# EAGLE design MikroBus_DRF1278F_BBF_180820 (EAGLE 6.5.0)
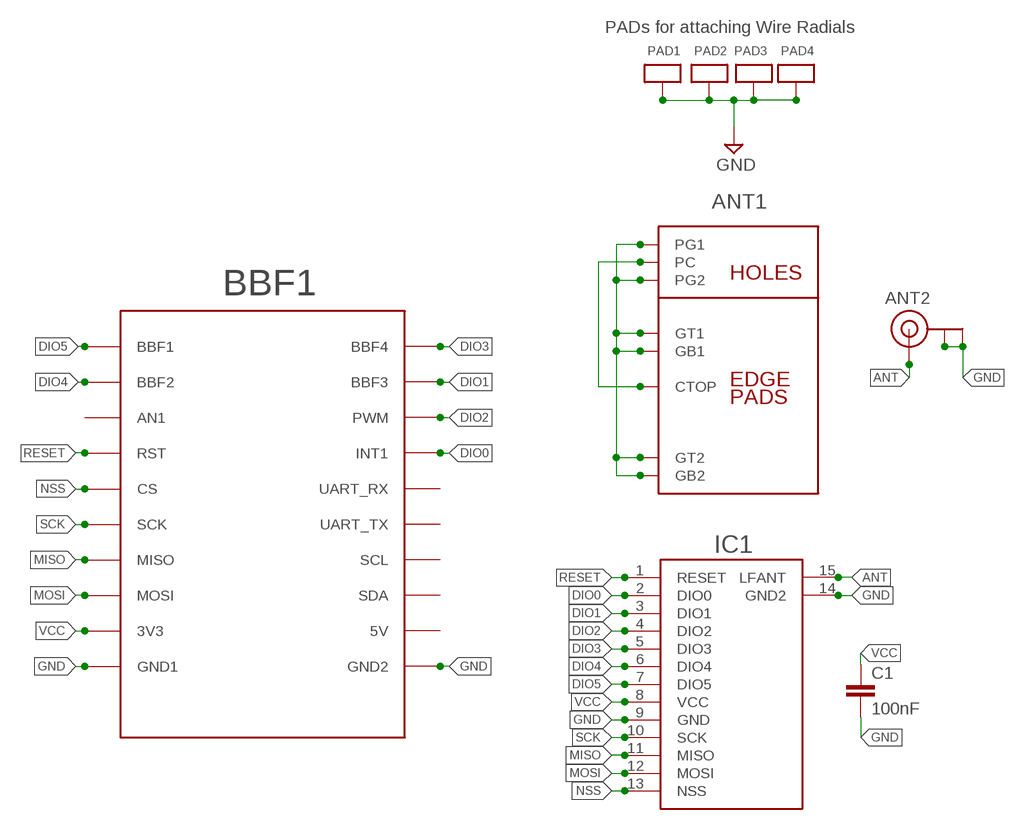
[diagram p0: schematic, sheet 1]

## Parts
ANT1  CUSTOMSMA  [CUSTOMSMA]
ANT2  ANTENNA_U.FL  [U.FL]
BBF1  BBFRIENDY2  [PCB_SOCKET_BBFRIENDLY2]
C1  100nF  C-EUC1206  [C1206]
IC1  DRF1278F  [DRF1278F]
PAD1  ANTPAD2  [ANTPAD2]
PAD2  ANTPAD2  [ANTPAD2]
PAD3  ANTPAD2  [ANTPAD2]
PAD4  ANTPAD2  [ANTPAD2]

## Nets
ANT: ANT1.CTOP ANT1.PC ANT2.3(SIGNAL) IC1.15(LFANT)
DIO0: BBF1.INT(INT1) IC1.2(DIO0)
DIO1: BBF1.BBF3 IC1.3(DIO1)
DIO2: BBF1.PWM IC1.4(DIO2)
DIO3: BBF1.BBF4 IC1.5(DIO3)
DIO4: BBF1.BBF2 IC1.6(DIO4)
DIO5: BBF1.BBF1 IC1.7(DIO5)
GND [VDD]: ANT1.G1 ANT1.G2 ANT1.GB1 ANT1.GB2 ANT1.GT1 ANT1.GT2 ANT2.1(GND) ANT2.2(GND) BBF1.GND1(GND2) BBF1.GND2(GND1) C1.2 IC1.9(GND) IC1.14(GND2) PAD1.P$1 PAD2.P$1 PAD3.P$1 PAD4.P$1
MISO: BBF1.MISO IC1.11(MISO)
MOSI: BBF1.MOSI IC1.12(MOSI)
NSS: BBF1.CS IC1.13(NSS)
RESET: BBF1.RST IC1.1(RESET)
SCK: BBF1.SCK IC1.10(SCK)
VCC [VDD]: BBF1.3V3 C1.1 IC1.8(VCC)
Unconnected: BBF1.5V BBF1.AN1 BBF1.RX(UART_RX) BBF1.SCL BBF1.SDA BBF1.TX(UART_TX)

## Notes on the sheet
- PADs for attaching Wire Radials
- BBF1

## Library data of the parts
ANT1 = con-coax:CUSTOMSMA
ANT2 = adafruit:ANTENNA_U.FL: U.FL Antenna Connector
BBF1 = My_Mikrobus:BBFRIENDY2
C1 = resistor:C-EU: CAPACITOR, European symbol
IC1 = LMA2:DRF1278F
PAD1-PAD4 = LMA2:ANTPAD2

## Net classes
0 default: width 0.152 mm
1 POWER: width 0.635 mm
2 VDD: width 0.635 mm

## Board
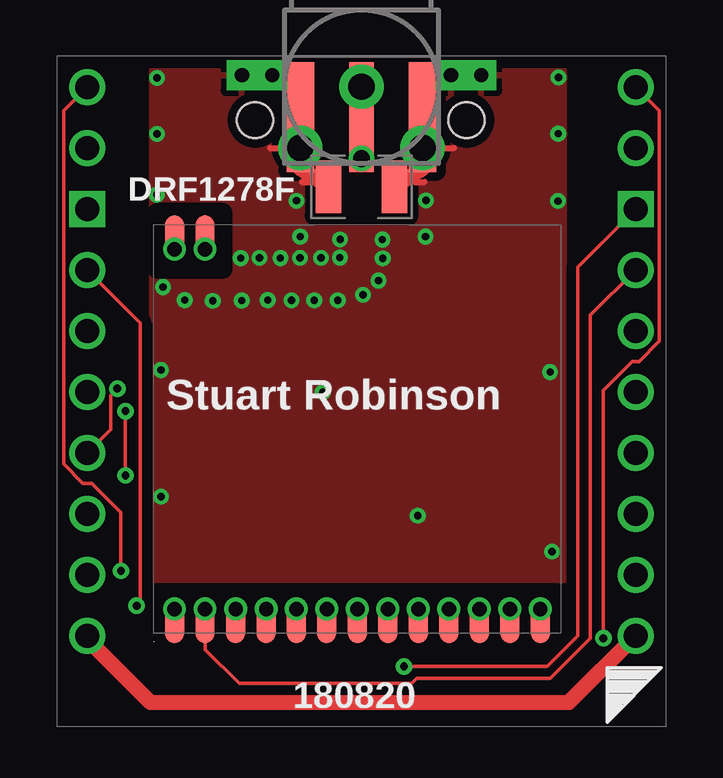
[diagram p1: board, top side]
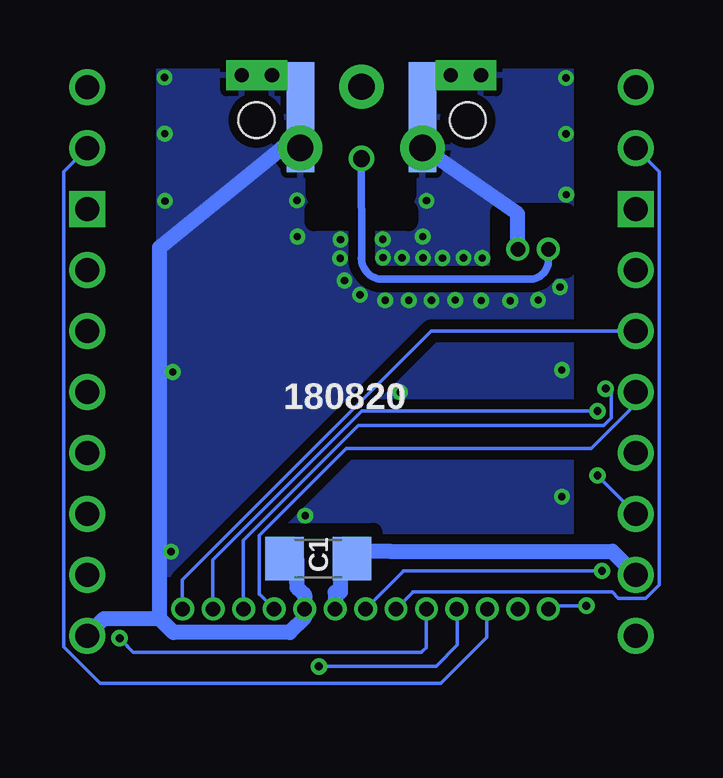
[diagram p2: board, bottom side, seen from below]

No outline drawn. Coordinates in mm, seen from the top.
Copper layers (1*16): Top 0.0356mm / dielectric 1.5011mm / Bottom 0.0356mm
Design rules "LaenPCBOrder *": minimum track width 6mil, minimum drill 13mil, track to track 6mil, track to pad 6mil, pad to pad 6mil, via to via 6mil, smd to smd 6mil, copper to edge 15mil, drill to drill 6mil, minimum pad ring 7mil, minimum via ring 7mil, stop-mask expansion 4mil, vias tented up to drill 1000mil, thermal gap 10mil
Holes 1.5 mm at 8.27,25.28 17.08,25.28
tRestrict: area 9.6,23.1 to 15.8,27.8; area 10.7,21.3 to 14.7,23.7; area 11.2,21.9 to 11.5,21.9; area 13.9,21.9 to 14.2,21.9; area 4.2,19.1 to 6.9,21.4; area 8.9,26.4 to 9.1,26.6
bRestrict: area 10.8,24.1 to 14.7,27.7; area 10.8,22.1 to 14.6,24.3; area 4.1,3.9 to 21.5,5.8; area 12.2,7.6 to 16.8,8.1; area 13.9,6 to 15.1,7.9; area 10.7,21 to 14.7,21.5; area 4.2,19.1 to 6.9,21.4; area 8.9,26.4 to 9.1,26.5

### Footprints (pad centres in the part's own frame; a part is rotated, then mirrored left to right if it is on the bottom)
CUSTOMSMA = smd 4.572 x 1.016: CTOP -1.27,0 | drill 1.1 pad 1.85: G1 -2.55,2.55; G2 -2.55,-2.55; PC 0,0 | smd 4.572 x 1.143 bottom: GB1 -1.27,2.54; GB2 -1.27,-2.54 | smd 4.572 x 1.143: GT1 -1.27,2.54; GT2 -1.27,-2.54
U.FL = smd 2.2 x 1.05: 1 0,1.375; 2 0,-1.375 | smd 0.8 x 1: 3 1.525,0
PCB_SOCKET_BBFRIENDLY2 = drill 1: 3V3 -11.43,5.08; 5V 11.43,5.08; BBF1 -11.43,25.4; BBF2 -11.43,22.86; BBF3 11.43,22.86; BBF4 11.43,25.4; CS -11.43,15.24; GND1 -11.43,2.54; GND2 11.43,2.54; INT 11.43,17.78; MISO -11.43,10.16; MOSI -11.43,7.62; RST -11.43,17.78; RX 11.43,15.24; SCK -11.43,12.7; SCL 11.43,10.16; SDA 11.43,7.62; TX 11.43,12.7 | drill 1 square: AN1 -11.43,20.32; PWM 11.43,20.32
C1206 = smd 1.6 x 1.8: 1 -1.4,0; 2 1.4,0
DRF1278F = drill 0.6 pad 0.85: 1 16.12,16; 2 14.85,16; 3 13.57,16; 4 12.3,16; 5 11.04,16; 6 9.77,16; 7 8.5,16; 8 7.23,16; 9 5.96,16; 10 4.69,16; 11 3.42,16; 12 2.15,16; 13 0.88,16; 14 14.85,1; 15 16.12,1 | smd 0.8 x 1.8: P$1 0.88,16.53; P$2 16.12,16.53; P$3 16.12,0.48; P$4 14.85,0.48; P$5 2.15,16.53; P$6 3.42,16.53; P$7 4.69,16.53; P$8 5.96,16.53; P$9 7.23,16.53; P$10 8.5,16.53; P$11 9.78,16.53; P$12 11.04,16.53; P$13 12.3,16.53; P$14 13.57,16.53; P$15 14.85,16.53
ANTPAD2 = drill 0.6 pad 1.27 square: P$1 0,0

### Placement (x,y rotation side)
ANT1  12.7,26.68 90 top
ANT2  12.7,22.5 90 top
BBF1  12.7,1.25 0 top
C1  14.5,7 180 bottom
IC1  21.03,20.9 180 top
PAD1  7.72,27.16 0 top
PAD2  8.98,27.16 0 top
PAD3  17.69,27.16 0 top
PAD4  16.43,27.16 0 top

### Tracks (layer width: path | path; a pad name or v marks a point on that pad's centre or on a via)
ANT  (via drill 0.7)
  Top 0.152: ANT2.3 ANT1.CTOP ANT1.PC
  Top 0.305: v12.7,23.68 12.69,24.15 ANT1.PC
  Bottom 0.305: IC1.15 4.91,19.43 arc90 5.69,18.65 11.82,18.65 arc90 12.7,19.53 12.69,19.53 v12.7,23.68
DIO0
  Top 0.152: BBF1.INT 22.24,17.15 22.24,3.67 20.57,2 20.5,2 15,2 14.8,1.8 8.47,1.8 7.6,1.8 6.2,3.2 6.2,4.88 IC1.2
DIO1
  Bottom 0.152: BBF1.BBF3 25.11,23.13 25.11,3.32 24.32,2.54 23.59,1.8 9.4,1.8 7.48,3.72 7.48,4.9 IC1.3
DIO2  (via drill 0.33 pad 0.69)
  Top 0.152: BBF1.PWM 21.72,19.16 21.72,3.78 20.44,2.51 v14.47,2.51
  Bottom 0.152: IC1.4 8.75,4.9 | 8.7,4.87 IC1.4 | v14.47,2.51 9.59,2.51 8.7,3.4 8.7,4.87 | 8.7,4.87 IC1.4
DIO3  (via drill 0.33 pad 0.69)
  Top 0.152: BBF1.BBF4 25.11,25.67 25.11,16.07 24.26,15.22 23.99,15.22 22.78,14.01 v22.78,3.68
  Bottom 0.152: 22.44,3.34 v22.78,3.68 22.2,3.1 10.2,3.1 10.1,3.2 10.01,3.29 10.01,4.9 IC1.5
DIO4
  Bottom 0.152: BBF1.BBF2 0.29,23.13 0.29,5.91 0.85,5.35 2,5.35 2.26,5.61 10.57,5.61 10.57,5.59 IC1.6
DIO5  (via drill 0.33 pad 0.69)
  Top 0.152: BBF1.BBF1 0.29,25.67 0.29,10.94 1.09,10.14 1.46,10.14 2.68,8.92 v2.68,6.49
  Bottom 0.152: v2.68,6.49 10.96,6.49 10.96,6.47 IC1.7
GND  (via drill 0.3)
  Top 0.254: 8.88,24.12 9.3,24.12 | 16.13,24.12 16.55,24.12 | 10.22,22.7 10.64,22.7 | 14.9,22.7 15.32,22.7
  Top 0.635: 10.16,24.86 ANT1.GB1 | 10.16,24.86 ANT1.G1 10.15,23.25 ANT2.1 | 10.16,24.86 10.2,24.82 | 15.07,24.67 ANT1.G2 | ANT1.G2 15.24,24.86 ANT1.GB2 | ANT2.2 15.25,23.25 ANT1.G2 | BBF1.GND1 1.27,3.63 3.9,1 21.34,1 BBF1.GND2
  Bottom 0.635: ANT1.G2 15.24,24.86 ANT1.GB2 | ANT1.GB1 10.16,24.86 ANT1.G1 6.19,21.38 6.19,19.92 6.2,19.92 IC1.14 | ANT1.G2 15.29,24.85 | 21.12,4.5 20.54,3.92 15.68,3.92 15.07,4.53 IC1.9 15.07,5.49 15.39,5.79 15.39,6.05 15.4,6.05 15.4,7 C1.2 | 21.12,4.5 21.12,18.95 21.12,19.97 16.03,24.12 ANT1.G2 | BBF1.GND2 23.42,4.5 21.12,4.5 | PAD3.P$1 PAD4.P$1
  other vias: 20.9,24.72 4.18,24.71 7.67,19.53 4.43,18.32 8.45,19.54 6.5,17.75 9.32,19.53 5.34,17.78 10.14,19.54 7.71,17.76 11.01,19.54 15.37,20.43 10.15,20.43 13.57,20.3 13.59,19.52 4.18,27.04 4.17,22.18 4.35,14.86 20.91,27.06 9.78,17.77 8.79,17.78 15.39,21.94 11.81,20.31 20.89,21.91 9.99,21.92 4.35,9.58 10.73,17.77 11.8,19.55 11.71,17.77 12.76,18 13.41,18.59 20.64,7.29 20.56,14.78 15.04,8.79 11.09,13.94
  pour Bottom (isolate 0.4): 3.85,27.4 21.25,27.4 21.25,3.7 3.85,3.7
  pour Top (isolate 0.4): 3.85,27.4 3.85,6 21.25,6 21.25,27.4
MISO  (via drill 0.33 pad 0.69)
  Top 0.152: BBF1.MISO 2.25,12.39 2.25,13.81 v2.53,14.09
  Bottom 0.152: v2.53,14.09 2.29,13.86 2.29,12.86 2.61,12.54 6.29,12.54 12.84,12.54 13.12,12.26 | 13.12,12.26 17.63,7.75 17.63,4.92 IC1.11 | 12.85,12.53 13.12,12.26
MOSI  (via drill 0.33 pad 0.69)
  Top 0.152: v2.87,13.15 v2.87,10.47
  Bottom 0.152: v2.87,13.15 12.69,13.15 18.9,6.94 18.9,4.92 IC1.12 | BBF1.MOSI v2.87,10.47
NSS
  Bottom 0.152: BBF1.CS 9.79,16.49 20.17,6.11 20.17,4.92 IC1.13
RESET  (via drill 0.33 pad 0.69)
  Top 0.152: BBF1.RST 3.47,16.83 3.47,5.18 v3.33,5.04
  Bottom 0.152: v3.33,5.04 4.79,5.04 arc-90 4.91,4.92 IC1.1
SCK
  Bottom 0.152: BBF1.SCK 1.27,13.45 3.13,11.59 13.34,11.59 16.96,7.96 16.96,5.5 16.94,5.5 IC1.10
VCC
  Bottom 0.635: BBF1.3V3 2.24,7.3 11.53,7.3 13.1,7.3 C1.1 13.58,7 13.58,5.6 13.8,5.6 IC1.8 13.83,4.93

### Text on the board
tPlace: DRF1278F | Stuart Robinson | 180820
bPlace: 180820 | C1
